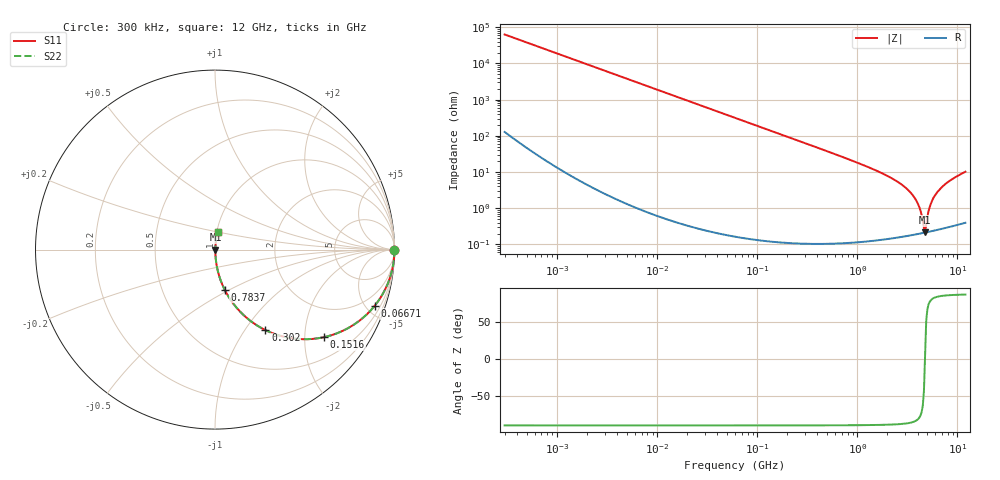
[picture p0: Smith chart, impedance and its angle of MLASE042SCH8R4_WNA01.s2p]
! MLASE042SCH8R4_WNA01  S-PARAMETER MODEL  ( General Type )
! Model Generated by TAIYO YUDEN Corporation (http://www.ty-top.com)
! Version 1.0
! TAIYO YUDEN Control No. 120810
! Copyright(c) 2012 TAIYO YUDEN CO.,LTD. All Rights Reserved.
! Product Description (link to TY-COMPAS)
! https://ds.yuden.co.jp/TYCOMPAS/or/detail?pn=MLASE042SCH8R4BWNA01&u=M
! Products Name : Multilayer Ceramic Capacitors
! Characteristics :
!  Capacitance : 8.4 pF , Rated Voltage : 16V , TCC : CH / C0H
!  Case Size : 0.4 x 0.2 / 0.016 x 0.008 [mm/inch] , Thickness : 0.2 / 0.008 [mm/inch]
!  (Conditions: Temperature = 25 degC , DC Bias Current/Voltage = 0A / 0V)
! External Node Assignments :
!  1  o---| |---o  2
! GND o---------o GND
! Frequency Range : 0.3MHz  -  12000MHz  [ 401 STEP ]
# MHz S RI R 50
! Freq[MHz].  S11 Real  S11 Imag  S21 Real  S21 Imag  S12 Real  S12 Imag  S22 Real  S22 Imag
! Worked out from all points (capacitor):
!   401 points, 300 kHz to 12 GHz, reference 50 ohm
!   read as one part in series: C = 8.4 pF near 316.3 kHz
!   lowest |Z| = 213 mohm at 4.748 GHz (marker M1)
!   series resonance near 4.736 GHz, so ESL is about 130 pH
!   S11 on the Smith chart (normalised r, x): 300 kHz: open; 66.71 MHz: 1.00, -5.68; 151.6 MHz: 1.00, -2.50; 302 MHz: 1.00, -1.25; 783.7 MHz: 1.00, -0.47; 12 GHz: 1.01, +0.20
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0.3  1 -0.00158  5.72e-06 0.00158  5.72e-06 0.00158  1 -0.00158
1.769972  0.9999 -0.00934  9.19e-05 0.00934  9.19e-05 0.00934  0.9999 -0.00934
10.44266  0.997 -0.0549  0.00305 0.0549  0.00305 0.0549  0.997 -0.0549
27.10171  0.9799 -0.1401  0.0201 0.1401  0.0201 0.1401  0.9799 -0.1401
60  0.9087 -0.2877  0.0913 0.2877  0.0913 0.2877  0.9087 -0.2877
66.70707  0.8896 -0.3132  0.1104 0.3132  0.1104 0.3132  0.8896 -0.3132
151.6462  0.609 -0.4875  0.391 0.4875  0.391 0.4875  0.609 -0.4875
301.9711  0.2812 -0.4488  0.7188 0.4488  0.7188 0.4488  0.2812 -0.4488
353.9943  0.2213 -0.4141  0.7787 0.4141  0.7787 0.4141  0.2213 -0.4141
783.7017  0.0533 -0.2224  0.9467 0.2224  0.9467 0.2224  0.0533 -0.2224
2088.533  0.00672 -0.0725  0.9933 0.0725  0.9933 0.0725  0.00672 -0.0725
2870.14  0.00337 -0.0416  0.9966 0.0416  0.9966 0.0416  0.00337 -0.0416
3547.679  0.00236 -0.0234  0.9976 0.0234  0.9976 0.0234  0.00236 -0.0234
4050.141  0.0021 -0.0126  0.9979 0.0126  0.9979 0.0126  0.0021 -0.0126
4270.516  0.00207 -0.00834  0.9979 0.00834  0.9979 0.00834  0.00207 -0.00834
4502.883  0.00207 -0.0041  0.9979 0.0041  0.9979 0.0041  0.00207 -0.0041
4747.894  0.00212 0.000206  0.9979 -0.000206  0.9979 -0.000206  0.00212 0.000206
4875.354  0.00216 0.00279  0.9978 -0.00279  0.9978 -0.00279  0.00216 0.00279
5420.343  0.00246 0.013  0.9975 -0.013  0.9975 -0.013  0.00246 0.013
6188.031  0.00315 0.0258  0.9968 -0.0258  0.9968 -0.0258  0.00315 0.0258
8064.993  0.00576 0.0528  0.9942 -0.0528  0.9942 -0.0528  0.00576 0.0528
12000  0.0141 0.1  0.9859 -0.1  0.9859 -0.1  0.0141 0.1
